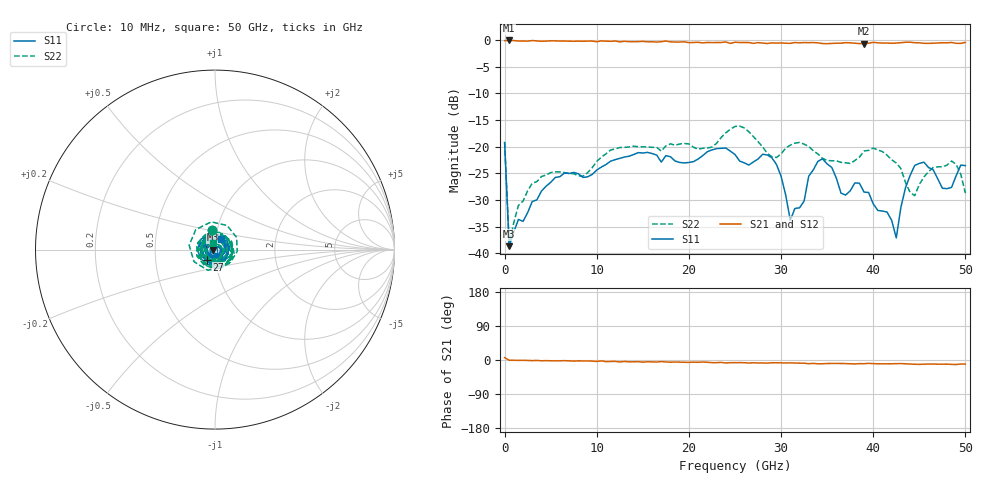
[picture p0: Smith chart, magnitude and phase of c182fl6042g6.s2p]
! 8/5/2019 2:18:48 PM
! Z:\MATT MILLER ENGINEERING\C182FL6042G6.S2P
! CHANNEL.1
! TR.MEASUREMENT
! CORRECTED.DATA
# GHZ S RI R 50.0
! FREQ.GHZ  S11RE  S11IM  S21RE  S21IM  S12RE  S12IM  S22RE  S22IM
!; PortSelection: Port_12
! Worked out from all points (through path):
!   101 points, 10 MHz to 50 GHz, reference 50 ohm
!   highest |S21| = -0.06 dB at 509.9 MHz (marker M1); lowest = -0.7 dB at 39 GHz (marker M2)
!   group delay of S21, straight-line fit = 628 fs
!   lowest |S11| = -38.7 dB at 509.9 MHz (marker M3), VSWR 1.02, Z = 48.8 - j0.0553 ohm
!   |S11| at or under -10 dB: start of sweep to end of sweep
!   |S22| runs from -38.3 to -16.1 dB; largest |S21 - S12| = 0.035
!   S11 on the Smith chart (normalised r, x): 10 MHz: 0.95, +0.21; 27 GHz: 0.91, -0.10; 50 GHz: 1.06, +0.12
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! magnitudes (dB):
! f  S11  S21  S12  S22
! 10 MHz  -19.2  -0.1  -0.1  -19.2
! 509.9 MHz  -38.7  -0.1  0.0  -38.3
! 1.51 GHz  -33.7  -0.2  -0.1  -31.0
! 3.009 GHz  -30.3  -0.1  -0.1  -26.9
! 6.509 GHz  -24.9  -0.2  -0.2  -24.9
! 8.508 GHz  -25.8  -0.2  -0.2  -25.5
! 11.51 GHz  -22.7  -0.2  -0.2  -20.6
! 17.01 GHz  -22.9  -0.3  -0.2  -20.8
! 25 GHz  -21.5  -0.4  -0.4  -16.2
! 27 GHz  -22.9  -0.6  -0.5  -18.1
! 29.5 GHz  -23.3  -0.6  -0.6  -22.0
! 31 GHz  -33.8  -0.6  -0.5  -19.7
! 33.5 GHz  -24.3  -0.5  -0.5  -20.8
! 34.5 GHz  -22.3  -0.6  -0.5  -22.2
! 36.5 GHz  -28.7  -0.6  -0.5  -22.9
! 39 GHz  -28.5  -0.7  -0.6  -20.8
! 42 GHz  -33.8  -0.6  -0.5  -22.5
! 42.5 GHz  -37.1  -0.5  -0.5  -23.1
! 43.5 GHz  -27.7  -0.4  -0.4  -26.7
! 44.5 GHz  -23.5  -0.5  -0.4  -29.2
! 48.5 GHz  -27.6  -0.4  -0.6  -22.7
! 50 GHz  -23.5  -0.4  -0.4  -28.7
